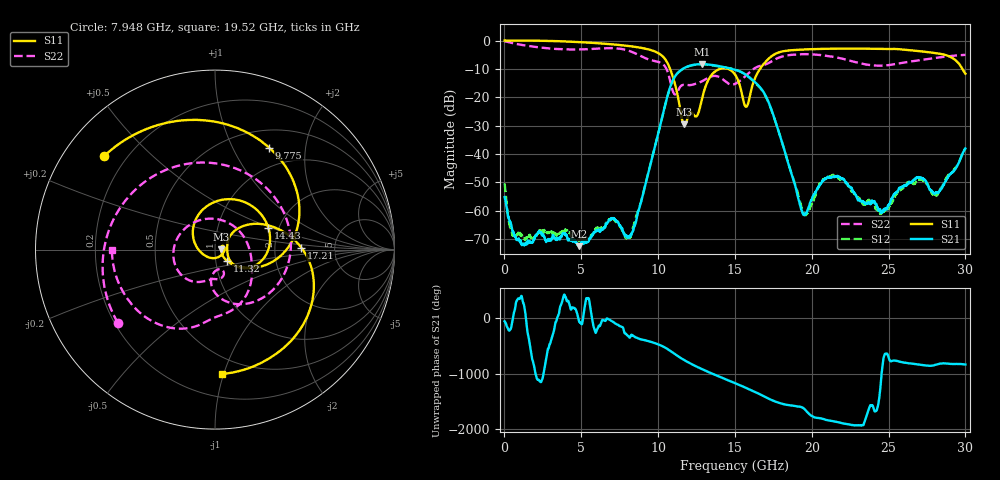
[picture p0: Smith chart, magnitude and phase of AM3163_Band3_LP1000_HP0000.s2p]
!Agilent Technologies,E8364B,MY43040894,A.07.50.67
!Agilent E8364B: A.07.50.67
!Date: Thursday, August 20, 2020 12:12:56
!Correction: S11(Full 2 Port(1,2))
!S21(Full 2 Port(1,2))
!S12(Full 2 Port(1,2))
!S22(Full 2 Port(1,2))
!S2P File: Measurements: S11, S21, S12, S22:
# Hz S  dB  R 50
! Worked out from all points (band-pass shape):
!   3201 points, 10 MHz to 30 GHz, reference 50 ohm
!   highest |S21| = -8.33 dB at 12.86 GHz (marker M1); lowest = -72.5 dB at 4.855 GHz (marker M2)
!   |S21| within 3 dB of the highest: 11.3 GHz to 15.48 GHz (4.189 GHz wide, 31.3 % of centre)
!   lowest |S11| = -29.6 dB at 11.72 GHz (marker M3), VSWR 1.07, Z = 53.4 + j0.234 ohm
!   |S11| at or under -10 dB: 10.78 GHz to 14.03 GHz (3.25 GHz wide, 26.2 % of centre); 14.54 GHz to 16.63 GHz (2.094 GHz wide, 13.4 % of centre); 29.8 GHz to end of sweep
!   |S22| runs from -19.0 to -0.3 dB; largest |S21 - S12| = 0.0093
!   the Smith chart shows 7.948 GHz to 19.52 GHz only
!   S11 on the Smith chart (normalised r, x): 7.948 GHz: 0.12, +0.36; 9.775 GHz: 0.72, +1.40; 11.32 GHz: 1.13, -0.14; 14.43 GHz: 1.76, +0.48; 17.21 GHz: 2.86, +0.08; 19.52 GHz: 0.37, -0.98
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1e7  0.02 -1.9  -55.21 -56.6  -50.39 -132.1  -0.29 -6.6
1.05965e9  -0.00 -29.0  -70.53 17.8  -68.72 99.8  -1.50 -84.4
2.362341e9  -0.07 -64.8  -67.57 -72.2  -67.23 152.1  -2.49 -166.0
4.855259e9  -0.56 -131.4  -72.53 -58.8  -70.72 -150.3  -3.17 61.6
5.014581e9  -0.60 -135.6  -71.09 -110.1  -70.26 134.0  -3.15 52.9
6.336016e9  -1.05 -171.5  -66.75 -53.2  -66.35 38.6  -2.77 -25.3
7.947978e9  -1.85 139.7  -69.08 61.5  -69.72 -40.5  -3.38 -143.0
8.978884e9  -2.66 101.3  -55.07 -28.2  -54.90 -25.7  -5.74 117.9
9.775494e9  -3.83 62.1  -37.88 -90.1  -37.91 -91.0  -7.25 25.8
1.000979e10  -4.43 47.6  -32.75 -113.9  -32.80 -114.6  -7.53 -3.0
1.132185e10  -20.68 -43.2  -11.19 26.8  -11.23 26.8  -17.34 -68.9
1.171547e10  -29.59 3.8  -9.65 -39.0  -9.72 -39.1  -15.62 -85.0
1.285884e10  -20.49 178.1  -8.33 159.9  -8.41 159.8  -14.37 -111.3
1.443332e10  -9.86 22.4  -9.52 -25.0  -9.55 -23.7  -14.66 118.3
1.5005e10  -11.97 -18.3  -10.30 -90.2  -10.24 -89.7  -15.30 33.1
1.574538e10  -23.33 5.6  -12.19 -180.0  -12.26 179.5  -12.23 -32.5
1.720739e10  -6.35 1.2  -21.96 -13.5  -22.14 -11.6  -7.91 -96.5
1.952224e10  -3.16 -87.0  -61.38 163.1  -61.62 149.2  -4.81 -179.6
2.000958e10  -3.03 -99.9  -55.94 35.9  -57.56 -112.8  -4.88 163.2
2.198705e10  -2.86 -146.4  -48.76 -93.7  -48.84 -93.5  -6.40 85.4
2.500479e10  -3.00 144.3  -58.20 7.4  -59.21 -73.5  -8.67 -72.6
3e10  -11.68 -28.7  -38.10 -116.7  -37.92 -117.3  -5.05 106.9
